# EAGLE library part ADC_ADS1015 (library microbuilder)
ADS1015 - 12-bit 4-Channel I2C ADC with Internal PGA VDD: 2.0-5.5V Sampling Rate: 3.3ksps Gain Settings: 2/3, 1, 2, 4, 8, 16 I2C Address: ADDR low = 1001000x, ADDR high = 1001001x Internal Comparator The ADS1015 includes an internal comparator that can be set to output a high-level on ALERT when the conversion results exceeeds a pre-defined upper level, and will deassert itself when the level falls below a pre-defined lower threshold level. It can also be set to windowed mode where the ALERT pin will be asserted if the data exceeds the upper threshold or falls below the lower threshold.
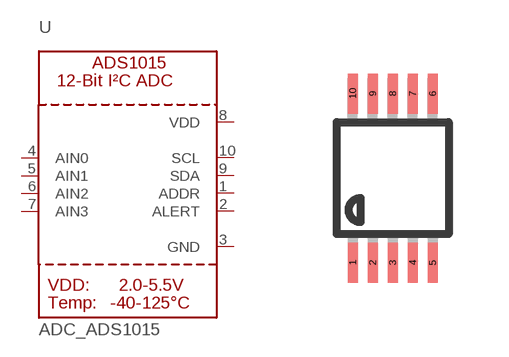
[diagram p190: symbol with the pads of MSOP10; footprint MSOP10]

Designator prefix U

## ADC_ADS1015  [MSOP10]
1  ADDR
2  ALERT
3  GND
4  AIN0
5  AIN1
6  AIN2
7  AIN3
8  VDD
9  SDA
10  SCL

## Footprint MSOP10 (pad centres in mm)
10-Lead Mini Small Outline Package [MSOP]
smd 0.25 x 1: 1 -1,-2.113; 2 -0.5,-2.113; 3 0,-2.113; 4 0.5,-2.113; 5 1,-2.113; 6 1,2.113; 7 0.5,2.113; 8 0,2.113; 9 -0.5,2.113; 10 -1,2.113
